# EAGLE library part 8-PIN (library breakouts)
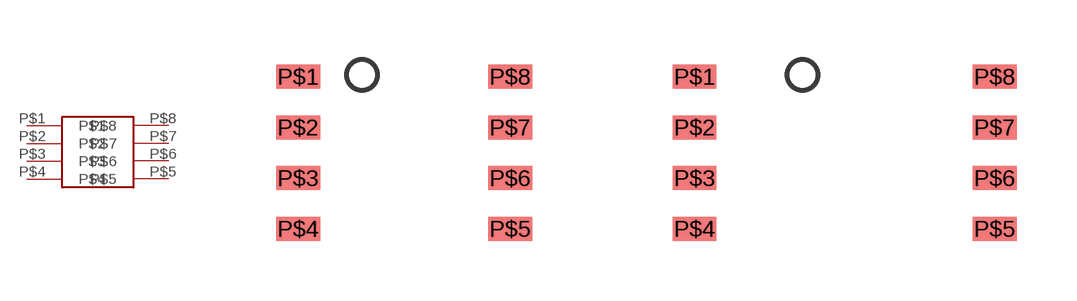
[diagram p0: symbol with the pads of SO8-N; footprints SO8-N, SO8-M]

Designator prefix -

## 8-PINSOIC-N  [SO8-N]
P$1  P$1
P$2  P$2
P$3  P$3
P$4  P$4
P$5  P$5
P$6  P$6
P$7  P$7
P$8  P$8

## 8-PINSOIC-W  [SO8-M]
Pads as for SO8-N

## 8-PINSOIC-NW  [SO8-NM]
Pads as for SO8-N

## 8-PINTSSOP  [TSSOP8]
Pads as for SO8-N

## Footprint SO8-N (pad centres in mm)
smd 1.1 x 0.6: P$1 -2.65,1.905; P$2 -2.65,0.635; P$3 -2.65,-0.635; P$4 -2.65,-1.905; P$5 2.65,-1.905; P$6 2.65,-0.635; P$7 2.65,0.635; P$8 2.65,1.905

## Footprint SO8-M (pad centres in mm)
smd 1.1 x 0.6: P$1 -3.75,1.905; P$2 -3.75,0.635; P$3 -3.75,-0.635; P$4 -3.75,-1.905; P$5 3.75,-1.905; P$6 3.75,-0.635; P$7 3.75,0.635; P$8 3.75,1.905

## Footprint SO8-NM (pad centres in mm)
smd 2.2 x 0.6: P$1 -3.2,1.905; P$2 -3.2,0.635; P$3 -3.2,-0.635; P$4 -3.2,-1.905; P$5 3.2,-1.905; P$6 3.2,-0.635; P$7 3.2,0.635; P$8 3.2,1.905

## Footprint TSSOP8 (pad centres in mm)
smd 1.45 x 0.35: P$1 -2.825,0.975; P$2 -2.825,0.325; P$3 -2.825,-0.325; P$4 -2.825,-0.975; P$5 2.825,-0.975; P$6 2.825,-0.325; P$7 2.825,0.325; P$8 2.825,0.975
